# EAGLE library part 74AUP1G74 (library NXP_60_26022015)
Low-power D-type flip-flop with set and reset; positive-edge trigger The 74AUP1G74 provides a low-power, low-voltage single positive-edge triggered D-type flip-flop with individual data (D), clock (CP), set (SD) and reset (RD) inputs and complementary Q and Q outputs. The SD and RD are asynchronous active LOW inputs and operate independently of the clock input. Information on the data input is transferred to the Q output on the LOW-to-HIGH transition of the clock pulse. The D input must be stable one set-up time prior to the LOW-to-HIGH clock transition for predictable operation. Schmitt trigger action at all inputs makes the circuit tolerant to slower input rise and fall times across the entire VCC range from 0.8 V to 3.6 V. This device ensures a very low static and dynamic power consumption across the entire VCC range from 0.8 V to 3.6 V. This device is fully specified for partial power-down applications using IOFF. The IOFF circuitry disables the output, preventing the damaging backflow current through the device when it is powered down. AAL Eindhoven MK
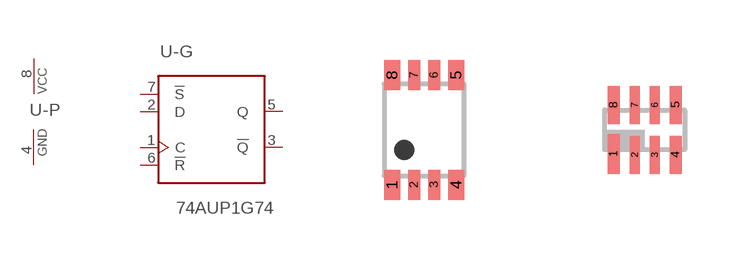
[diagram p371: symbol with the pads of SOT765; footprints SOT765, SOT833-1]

Designator prefix U; gates -G=D-FLIPFLOP_SR -P=PWRN

## 74AUP1G74DC  [SOT765]
1  -G:C  in
2  -G:D  in
3  -G:!Q  out
4  -P:GND  pwr
5  -G:Q  out
6  -G:!R  in
7  -G:!S  in
8  -P:VCC  pwr

## 74AUP1G74GT  [SOT833-1]
Pads as for SOT765

## 74AUP1G74GF  [SOT1089-1]
Pads as for SOT765

## 74AUP1G74GD  [SOT996-2/3]
Pads as for SOT765

## 74AUP1G74GM  [SOT902-1/2/3]
1  -G:!S  in
2  -G:!R  in
3  -G:Q  out
4  -P:GND  pwr
5  -G:!Q  out
6  -G:D  in
7  -G:C  in
8  -P:VCC  pwr

## 74AUP1G74GS  [SOT1203]
Pads as for SOT765

## Footprint SOT765 (pad centres in mm)
SOT765 VSSOP8: plastic very thin shrink small outline package; 8 leads; body width 2.3 mm JEDEC: MO-187 IEC: -- JEITA: --
smd 0.4 x 0.75: 1 -0.8,-1.375; 4 0.8,-1.375; 5 0.8,1.375; 8 -0.8,1.375
smd 0.3 x 0.75: 2 -0.25,-1.375; 3 0.25,-1.375; 6 0.25,1.375; 7 -0.25,1.375

## Footprint SOT833-1 (pad centres in mm)
SOT833-1 XSON8: plastic extremely thin small outline package; no leads; 8 terminals; body 1 x 1.95 x 0.5 mm JEDEC: MO-252 IEC: -- JEITA: --
smd 0.3 x 1: 1 -0.775,-0.6
smd 0.25 x 0.95: 2 -0.25,-0.625; 3 0.25,-0.625; 6 0.25,0.625; 7 -0.25,0.625
smd 0.3 x 0.95: 4 0.775,-0.625; 5 0.775,0.625; 8 -0.775,0.625

## Footprint SOT1089-1 (pad centres in mm)
SOT1089-1 XSON8: plastic, extremely thin small outline package; no leads; 8 terminals; body 1 x 1.35 x 0.5 mm JEDEC: -- IEC: -- JEITA: --
smd 0.15 x 0.5: 1 -0.525,-0.35; 2 -0.175,-0.35; 3 0.175,-0.35; 4 0.525,-0.35; 5 0.525,0.35; 6 0.175,0.35; 7 -0.175,0.35; 8 -0.525,0.35

## Footprint SOT996-2/3 (pad centres in mm)
SOT996-2/3 XSON8U: plastic extremely thin small outline package; no leads;8 terminals; UTLP based; body 3 x 2 x 0.5 mm JEDEC: IEC: -- JEITA: --
smd 0.25 x 1.1: 1 -0.75,-1.45
smd 0.25 x 1: 2 -0.25,-1.5; 3 0.25,-1.5; 4 0.75,-1.5; 5 0.75,1.5; 6 0.25,1.5; 7 -0.25,1.5; 8 -0.75,1.5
